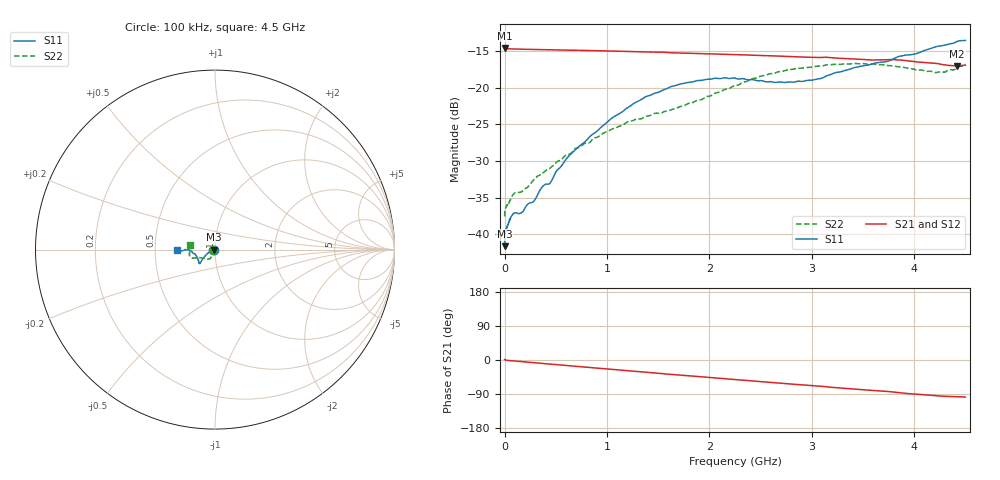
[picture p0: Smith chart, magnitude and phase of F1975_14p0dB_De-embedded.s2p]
! Integrated Device Technology
! Corporate Headquarters
! 6024 Silver Creek Valley Road
! San Jose, CA 95138  USA
! Phone:  1-408-284-8200
! Toll Free:  1-800-223-1366
! Webpage:  http://www.idt.com/
! Timing and RF Division
! 515 Groton Road, Suite 102
! Westford, MA 01886-6024
! Device:  F1975
! Description: 6-bit, 75 ohm, 0.5 dB Digital Step Attenuator
! Frequency:  5.0 MHz -  3.00 GHz
! Package:  4x4 mm QFN Plastic Package: 20 pin
! Ports:  2 RF, 11 DC
!  Pin  1  = D5 (16 dB)
!  Pin  2  = RF1  =  Port 1
!  Pin  3  = Serial Data In (DATA)
!  Pin  4  = Serial Clock (CLK)
!  Pin  5  = Serial Latch Enable (LE)
!  Pin  6  = VDD
!  Pin  7  = NC
!  Pin  8  = NC
!  Pin  9  = NC
!  Pin 10  = GND
!  Pin 11  = GND
!  Pin 12  = NC
!  Pin 13  = VMODE
!  Pin 14  = RF2  =  Port 2
!  Pin 15  = D4 (8 dB)
!  Pin 16  = D3 (4 dB)
!  Pin 17  = D2 (2 dB)
!  Pin 18  = NC
!  Pin 19  = D1 (1 dB)
!  Pin 20  = D0 (0.5 dB)
! State:  28
! Atten State:  14.0 dB
! Voltage:  +3.30 Volts
! Current:  0.594 mA
! Data:  The device was measured on a F1975 evaluation board which has
!  individual transmission lines to the RF pins.  Data was collected
!  using a calibrated network analyzer.  The evaluation board was
!  de-embedded using Automatic Fixture Removal (AFR).
!  The reference plane is the edge of the package pin.
! Misc:
!  Action Tracker AT0415
! Date Measured:  2018-02-08
! Date:  2018-03-26  MJV
! Note:
!  Integrated Device Technology supplies this data as a sample of measured
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# GHz S dB R 75
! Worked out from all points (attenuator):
!   291 points, 100 kHz to 4.5 GHz, reference 75 ohm
!   highest |S21| = -14.60 dB at 100 kHz (marker M1); lowest = -17.0 dB at 4.42 GHz (marker M2)
!   lowest |S11| = -41.6 dB at 100 kHz (marker M3), VSWR 1.02, Z = 73.8 - j0.019 ohm
!   |S11| at or under -10 dB: start of sweep to end of sweep
!   |S22| runs from -37.6 to -16.7 dB; largest |S21 - S12| = 0.00016
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0.0001  -41.62 -179.1  -14.60 1.2  -14.61 1.2  -37.58 -178.5
0.0005  -40.71 -176.3  -14.62 1.1  -14.63 1.1  -37.32 -177.8
0.002  -40.18 -176.7  -14.64 0.8  -14.65 0.8  -36.86 -176.3
0.011  -39.48 -174.7  -14.68 -0.5  -14.68 -0.5  -36.34 -173.8
0.08  -37.27 -167.5  -14.73 -2.2  -14.73 -2.2  -34.61 -162.0
0.16  -37.08 -163.8  -14.76 -4.2  -14.76 -4.2  -34.25 -146.7
0.28  -35.59 -162.7  -14.80 -7.0  -14.79 -7.0  -32.63 -136.2
0.36  -33.66 -163.1  -14.82 -8.9  -14.82 -8.9  -31.70 -128.1
0.44  -33.09 -160.6  -14.84 -10.7  -14.84 -10.7  -31.04 -122.6
0.6  -29.77 -158.9  -14.88 -14.4  -14.88 -14.4  -29.18 -119.2
0.76  -27.66 -153.4  -14.92 -18.1  -14.92 -18.1  -27.84 -117.6
1.06  -24.05 -147.8  -15.02 -25.1  -15.01 -25.1  -25.59 -117.4
1.38  -21.22 -143.3  -15.14 -32.3  -15.14 -32.3  -23.91 -124.0
1.52  -20.54 -140.8  -15.16 -35.4  -15.16 -35.4  -23.50 -127.8
1.88  -19.05 -137.7  -15.35 -43.4  -15.35 -43.4  -21.73 -142.9
2.26  -18.75 -139.7  -15.50 -51.7  -15.50 -51.7  -19.70 -154.3
2.58  -19.20 -149.2  -15.65 -58.7  -15.65 -58.7  -18.15 -157.6
3.02  -18.93 -166.2  -15.87 -68.0  -15.87 -68.0  -17.15 -161.4
3.76  -16.32 -179.0  -16.18 -83.5  -16.18 -83.5  -17.01 -175.0
4.2  -14.48 -177.9  -16.68 -93.9  -16.68 -93.9  -17.94 173.4
4.42  -13.71 -177.1  -17.03 -96.7  -17.03 -96.7  -17.25 170.2
4.5  -13.57 -178.9  -16.94 -97.9  -16.94 -97.9  -16.81 169.0
